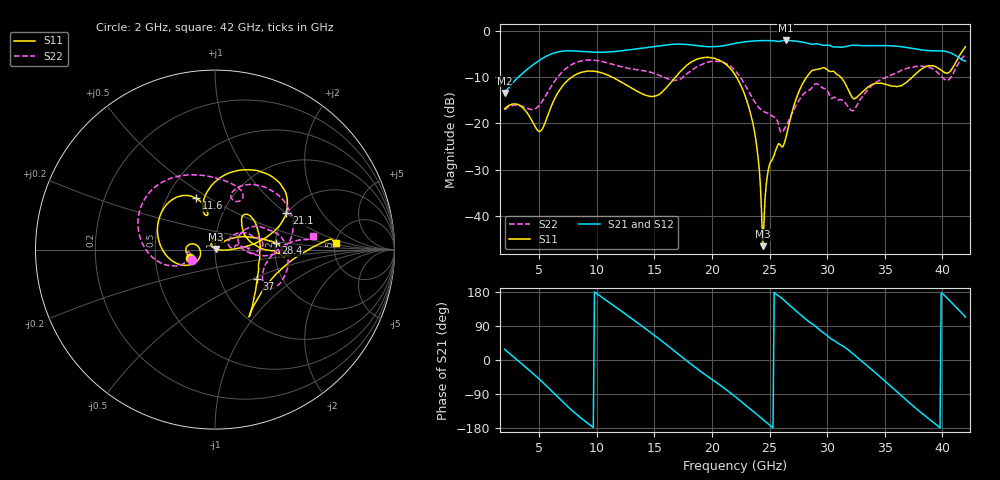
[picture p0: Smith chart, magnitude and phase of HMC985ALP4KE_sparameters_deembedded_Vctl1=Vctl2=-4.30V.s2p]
!s2p File: Measurements: S11, S21, S12, S22
# GHz S dB R 50.0
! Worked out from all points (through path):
!   401 points, 2 GHz to 42 GHz, reference 50 ohm
!   highest |S21| = -2.07 dB at 26.4 GHz (marker M1); lowest = -13.4 dB at 2 GHz (marker M2)
!   lowest |S11| = -46.5 dB at 24.4 GHz (marker M3), VSWR 1.01, Z = 50.3 + j0.327 ohm
!   |S11| at or under -10 dB: start of sweep to 7.825 GHz; 22.13 GHz to 28.22 GHz (6.091 GHz wide, 24.2 % of centre); 31.17 GHz to 37.39 GHz (6.218 GHz wide, 18.1 % of centre)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
!   |S22| runs from -22.0 to -5.2 dB; largest |S21 - S12| = 0.00068
!   S11 on the Smith chart (normalised r, x): 2 GHz: 0.76, -0.07; 11.6 GHz: 0.70, +0.44; 21.1 GHz: 1.98, +1.00; 28.4 GHz: 2.01, +0.17; 37 GHz: 1.50, -0.53; 42 GHz: 5.03, +0.68
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2  -16.80 -161.9  -13.45 28.2  -13.45 28.2  -17.10 -155.7
5  -21.74 -173.7  -6.39 -50.3  -6.39 -50.3  -16.11 -160.4
6.3  -14.89 -150.9  -4.77 -88.5  -4.77 -88.5  -11.01 -162.1
8.7  -8.94 150.0  -4.45 -154.8  -4.45 -154.8  -6.46 150.9
11.6  -10.34 110.1  -4.45 140.6  -4.45 140.7  -7.39 103.1
13.6  -13.18 101.4  -3.84 96.7  -3.85 96.7  -8.44 75.3
15.4  -13.76 106.4  -3.24 55.9  -3.24 55.9  -9.58 62.0
17.9  -7.26 79.8  -2.95 -4.3  -2.95 -4.3  -9.13 72.0
21.1  -7.02 27.1  -3.15 -75.1  -3.15 -75.1  -6.91 15.5
22  -9.46 16.6  -2.71 -96.4  -2.72 -96.4  -8.54 0.1
23.6  -20.60 0.8  -2.19 -136.2  -2.19 -136.2  -14.88 -4.0
24.4  -46.54 43.6  -2.09 -156.3  -2.09 -156.3  -17.31 7.9
25  -28.82 128.9  -2.12 -171.6  -2.12 -171.6  -17.96 11.7
26.4  -23.25 41.6  -2.07 153.6  -2.07 153.6  -20.68 33.5
28.4  -9.38 6.2  -2.74 101.6  -2.74 101.5  -12.88 17.7
28.7  -8.57 1.2  -2.88 95.4  -2.88 95.4  -12.18 15.9
32.4  -14.67 29.4  -3.09 12.0  -3.09 12.0  -16.85 26.0
33.9  -11.59 48.5  -3.21 -26.1  -3.21 -26.1  -11.77 30.2
35.4  -11.76 18.2  -3.21 -66.1  -3.20 -66.1  -9.74 18.9
37  -10.89 -34.6  -3.62 -109.2  -3.62 -109.2  -8.06 4.2
39.8  -8.30 -56.6  -4.31 -179.2  -4.31 -179.1  -9.52 -35.1
42  -3.43 3.2  -6.48 113.2  -6.49 113.2  -5.19 7.8
